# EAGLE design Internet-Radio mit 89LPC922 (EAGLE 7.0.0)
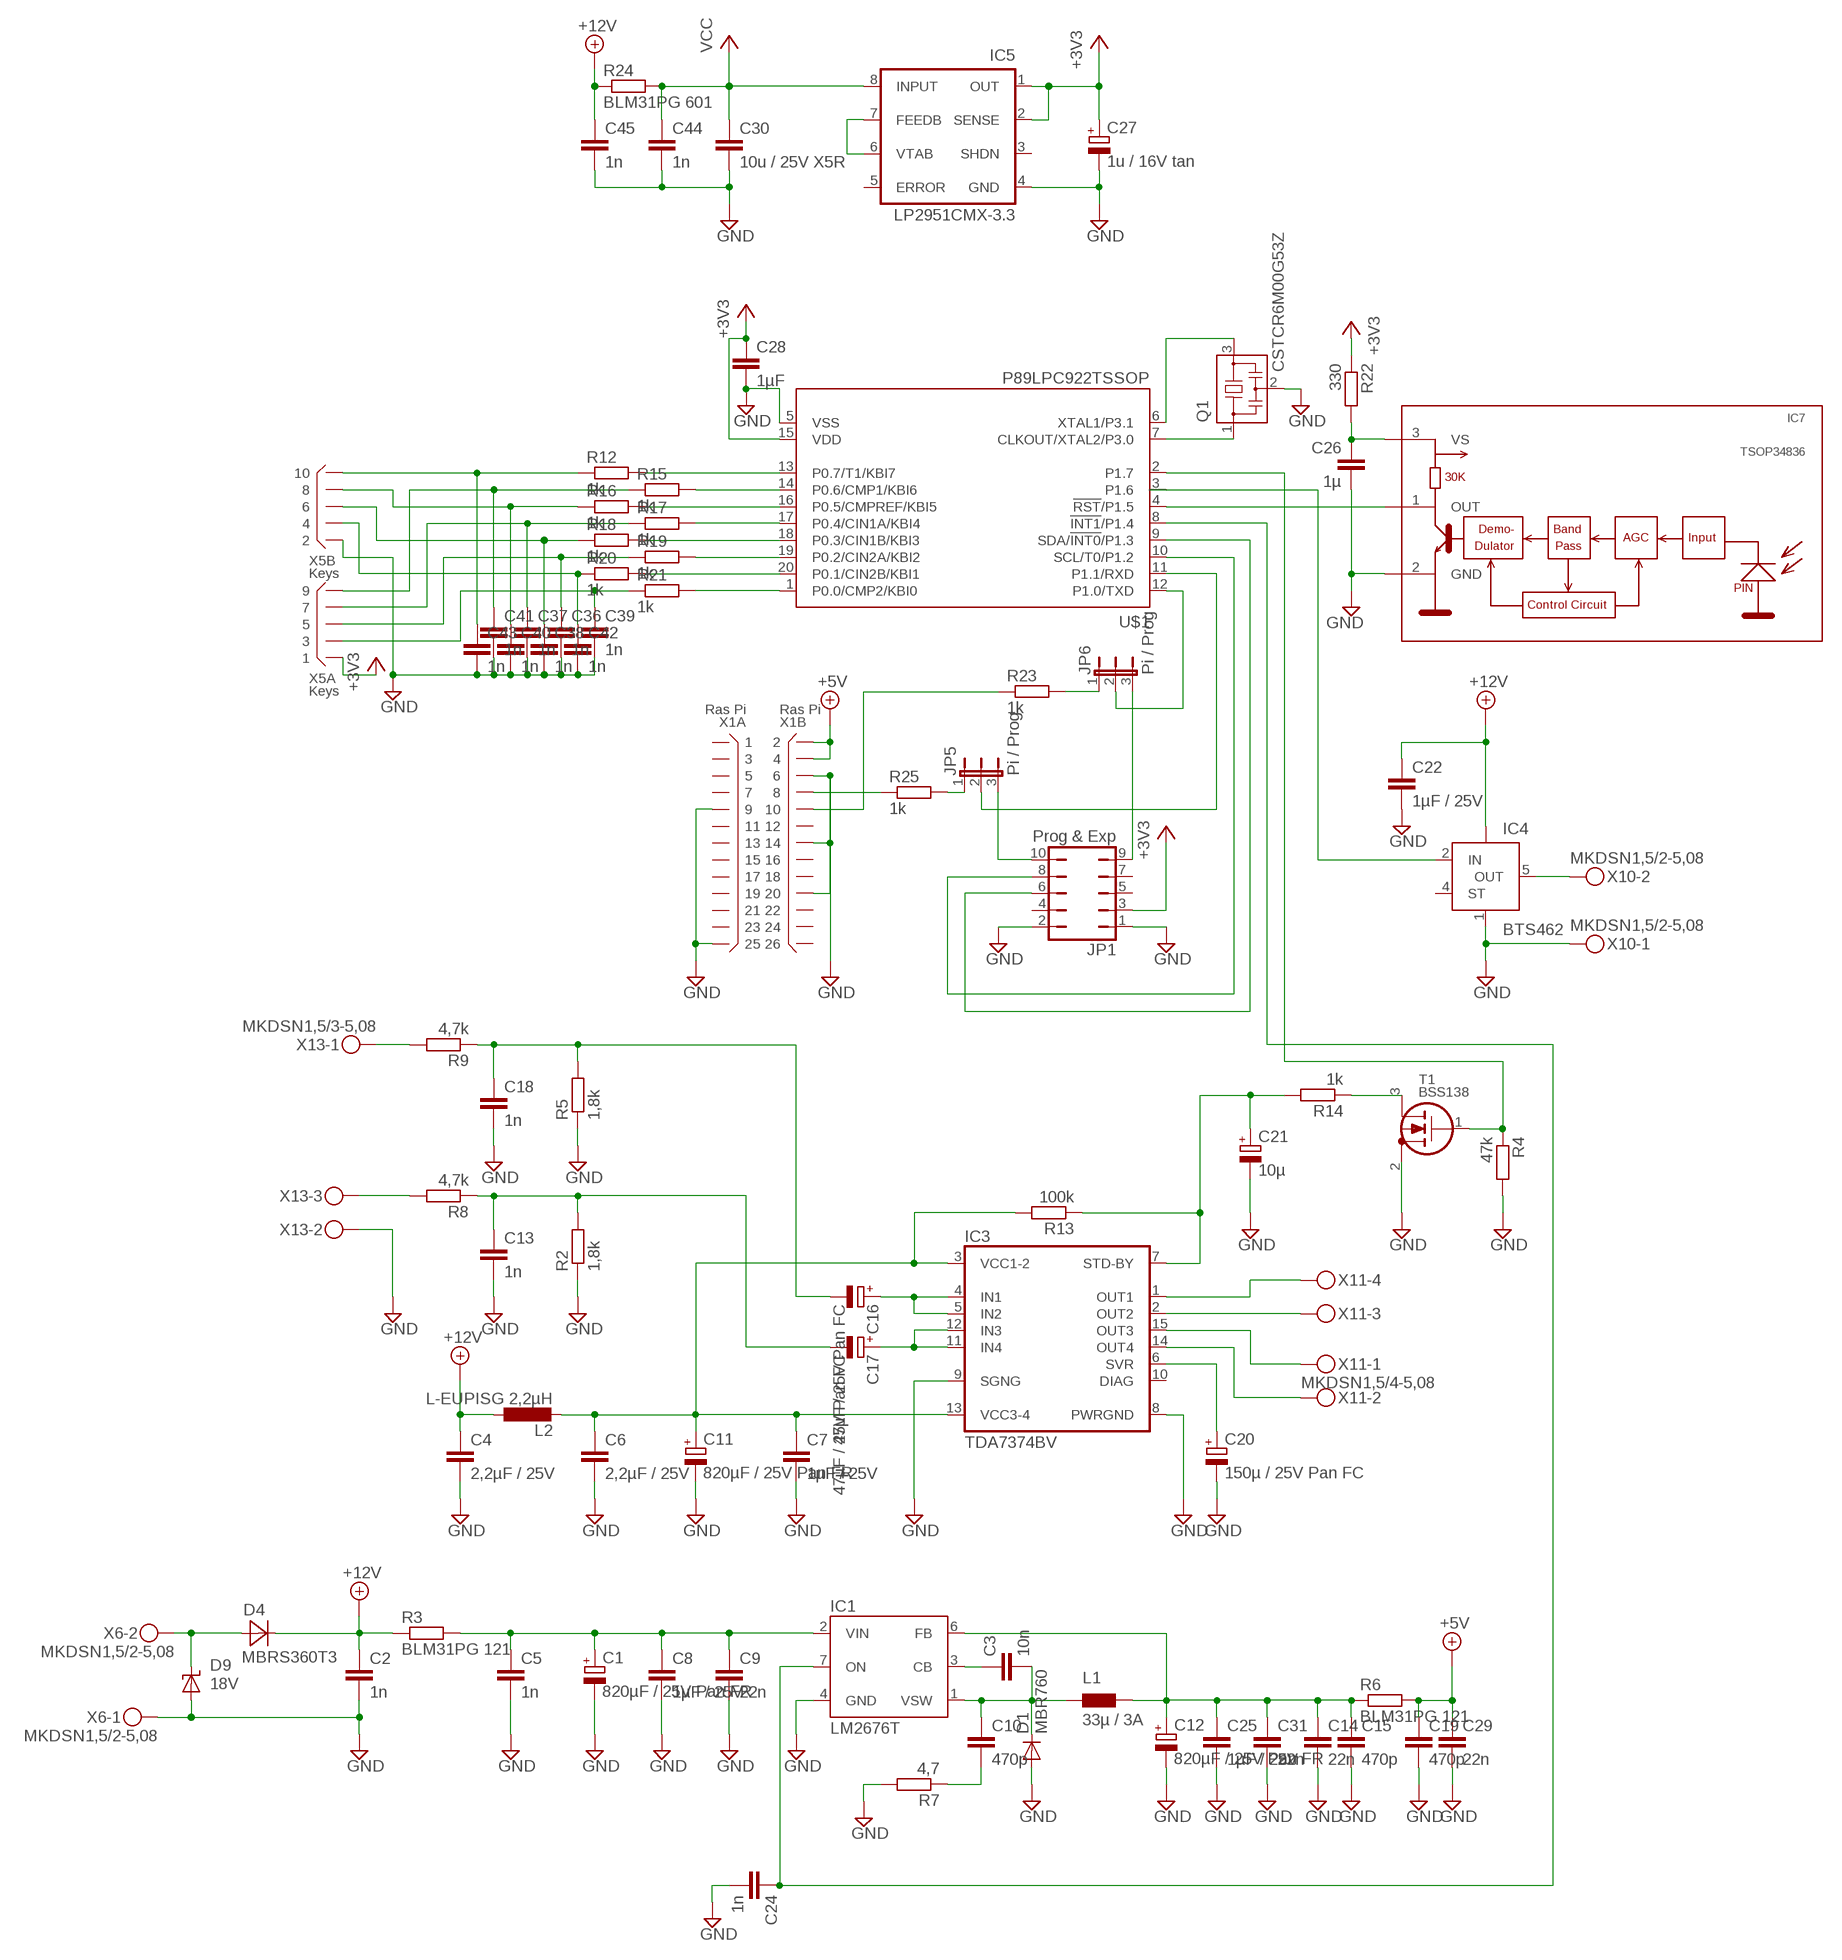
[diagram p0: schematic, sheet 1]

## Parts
C1  820µF / 25V Pan FR  CPOL-EUTT5D10  [TT5D10]
C2  1n  C-EUC0805  [C0805]
C3  10n  C-EUC0805  [C0805]
C4  2,2µF / 25V  C-EUC0805  [C0805]
C5  1n  C-EUC0805  [C0805]
C6  2,2µF / 25V  C-EUC0805  [C0805]
C7  1µF / 25V  C-EUC0805  [C0805]
C8  1µF / 25V  C-EUC0805  [C0805]
C9  22n  C-EUC0805  [C0805]
C10  470p  C-EUC0805  [C0805]
C11  820µF / 25V Pan FR  CPOL-EUTT5D10  [TT5D10]
C12  820µF / 25V Pan FR  CPOL-EUTT5D10  [TT5D10]
C13  1n  C-EUC0805  [C0805]
C14  22n  C-EUC0805  [C0805]
C15  470p  C-EUC0805  [C0805]
C16  47µF / 25V Pan FC  CPOL-EUE2.5-5  [E2,5-5]
C17  47µF / 25V Pan FC  CPOL-EUE2.5-5  [E2,5-5]
C18  1n  C-EUC0805  [C0805]
C19  470p  C-EUC0805  [C0805]
C20  150µ / 25V Pan FC  CPOL-EUE3.5-8  [E3,5-8]
C21  10µ  CPOL-EUE2.5-5  [E2,5-5]
C22  1µF / 25V  C-EUC0805  [C0805]
C24  1n  C-EUC0805  [C0805]
C25  1µF / 25V  C-EUC0805  [C0805]
C26  1µ  C-EUC0805  [C0805]
C27  1u / 16V tan  CPOL-EUCT3216  [CT3216]
C28  1µF  C-EUC0805  [C0805]
C29  22n  C-EUC0805  [C0805]
C30  10u / 25V X5R  C-EUC1206  [C1206]
C31  22n  C-EUC0805  [C0805]
C36  1n  C-EUC0603  [C0603]
C37  1n  C-EUC0603  [C0603]
C38  1n  C-EUC0603  [C0603]
C39  1n  C-EUC0603  [C0603]
C40  1n  C-EUC0603  [C0603]
C41  1n  C-EUC0603  [C0603]
C42  1n  C-EUC0603  [C0603]
C43  1n  C-EUC0603  [C0603]
C44  1n  C-EUC0805  [C0805]
C45  1n  C-EUC0805  [C0805]
D1  MBR760  DIODE-TO220V  [TO220ACS]
D4  MBRS360T3  [SMC]
D9  18V  SUPPRESSOR-SMBJ  [SMBJ]
IC1  LM2676T  [TO220-7]
IC3  TDA7374BV  [MULTIWATT-15V]
IC4  BTS462  BTS428L2  [TO252-5-11]
IC5  LP2951CMX-3.3  [SO-08]
IC7  TSOP34836  [TSOP348]
JP1  Prog & Exp  JP5Q  [JP5Q]
JP5  Pi / Prog  JP2E  [JP2]
JP6  Pi / Prog  JP2E  [JP2]
L1  33µ / 3A  PIS4728  [PIS4728]
L2  L-EUPISG 2,2µH  L-EUPISG  [PISG]
Q1  CSTCR6M00G53Z  [CSTCR6M]
R2  1,8k  R-EU_R1206  [R1206]
R3  BLM31PG 121  R-EU_R1206  [R1206]
R4  47k  R-EU_R1206  [R1206]
R5  1,8k  R-EU_R1206  [R1206]
R6  BLM31PG 121  R-EU_R1206  [R1206]
R7  4,7  R-EU_R1206  [R1206]
R8  4,7k  R-EU_R1206  [R1206]
R9  4,7k  R-EU_R1206  [R1206]
R12  1k  R-EU_R1206  [R1206]
R13  100k  R-EU_R1206  [R1206]
R14  1k  R-EU_R1206  [R1206]
R15  1k  R-EU_R1206  [R1206]
R16  1k  R-EU_R1206  [R1206]
R17  1k  R-EU_R1206  [R1206]
R18  1k  R-EU_R1206  [R1206]
R19  1k  R-EU_R1206  [R1206]
R20  1k  R-EU_R1206  [R1206]
R21  1k  R-EU_R1206  [R1206]
R22  330  R-EU_R1206  [R1206]
R23  1k  R-EU_R1206  [R1206]
R24  BLM31PG 601  R-EU_R1206  [R1206]
R25  1k  R-EU_R1206  [R1206]
T1  BSS138  [SOT23]
U$1  P89LPC922TSSOP  [SOT360]
X1  Ras Pi  X13X2  [X26N-IDC]
X5  Keys  X05X2  [X10N-IDC]
X6  MKDSN1,5/2-5,08  [MKDSN1,5/2-5,08]
X10  MKDSN1,5/2-5,08  [MKDSN1,5/2-5,08]
X11  MKDSN1,5/4-5,08  [MKDSN1,5/4-5,08]
X13  MKDSN1,5/3-5,08  [MKDSN1,5/3-5,08]

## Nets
+3V3: C27.+ C28.1 IC5.1(OUT) IC5.2(SENSE) JP1.3 R22.1 U$1.15(VDD) X5.1
+5V: C19.1 C29.1 R6.2 X1.2 X1.4
+12V: C2.1 C4.1 C22.1 C45.1 D4.C IC4.TAB(VBB) L2.1 R3.1 R24.1
GND: C1.- C2.2 C4.2 C5.2 C6.2 C7.2 C8.2 C9.2 C11.- C12.- C13.2 C14.2 C15.2 C18.2 C19.2 C20.- C21.- C22.2 C24.2 C25.2 C26.2 C27.- C28.2 C29.2 C30.2 C31.2 C36.2 C37.2 C38.2 C39.2 C40.2 C41.2 C42.2 C43.2 C44.2 C45.2 D1.A D9.A IC1.4(GND) IC3.8(PWRGND) IC3.9(SGNG) IC4.1(GND) IC5.4(GND) IC7.2(GND) JP1.1 JP1.2 Q1.2 R2.1 R4.2 R5.1 R7.2 T1.2(S) U$1.5(VSS) X1.6 X1.9 X1.14 X1.20 X1.25 X5.2 X6.1 X10.1 X13.2
N$1: C1.+ C5.1 C8.1 C9.1 IC1.2(VIN) R3.2
N$2: C3.2 C10.1 D1.C IC1.1(VSW) L1.P$1
N$3: IC3.1(OUT1) X11.4
N$4: C3.1 IC1.3(CB)
N$5: IC3.2(OUT2) X11.3
N$6: IC3.15(OUT3) X11.1
N$7: IC3.14(OUT4) X11.2
N$8: C6.1 C7.1 C11.+ IC3.3(VCC1-2) IC3.13(VCC3-4) L2.2 R13.2
N$9: D4.A D9.C X6.2
N$10: C20.+ IC3.6(SVR)
N$11: JP1.10 JP5.3
N$12: C16.- C18.1 R5.2 R9.1
N$13: R9.2 X13.1
N$14: C13.1 C17.- R2.2 R8.1
N$15: C10.2 R7.1
N$16: R8.2 X13.3
N$17: C12.+ C14.1 C15.1 C25.1 C31.1 IC1.6(FB) L1.P$2 R6.1
N$18: C21.+ IC3.7(STD-BY) R13.1 R14.2
N$19: Q1.3 U$1.6(XTAL1/P3.1)
N$20: IC4.5(OUT) X10.2
N$21: Q1.1 U$1.7(CLKOUT/XTAL2/P3.0)
N$22: R21.2 U$1.1(P0.0/CMP2/KBI0)
N$23: R14.1 T1.3(D)
N$24: C16.+ IC3.4(IN1) IC3.5(IN2)
N$25: R4.1 T1.1(G) U$1.2(P1.7)
N$26: C17.+ IC3.11(IN4) IC3.12(IN3)
N$27: R19.2 U$1.19(P0.2/CIN2A/KBI2)
N$28: C24.1 IC1.7(ON) U$1.8(!INT1!/P1.4)
N$29: JP5.2 U$1.11(P1.1/RXD)
N$30: R17.2 U$1.17(P0.4/CIN1A/KBI4)
N$31: R15.2 U$1.14(P0.6/CMP1/KBI6)
N$32: R12.2 U$1.13(P0.7/T1/KBI7)
N$33: IC7.1(OUT) U$1.4(!RST!/P1.5)
N$34: R16.2 U$1.16(P0.5/CMPREF/KBI5)
N$35: R18.2 U$1.18(P0.3/CIN1B/KBI3)
N$36: R20.2 U$1.20(P0.1/CIN2B/KBI1)
N$37: JP6.2 U$1.12(P1.0/TXD)
N$38: JP1.8 U$1.10(SCL/T0/P1.2)
N$39: JP1.6 U$1.9(SDA/!INT0!/P1.3)
N$40: C26.1 IC7.3(VS) R22.2
N$41: IC5.6(VTAB) IC5.7(FEEDB)
N$42: C38.1 R18.1 X5.6
N$43: C36.1 R19.1 X5.5
N$44: C42.1 R20.1 X5.4
N$45: C39.1 R21.1 X5.3
N$46: C43.1 R12.1 X5.10
N$47: C41.1 R15.1 X5.9
N$48: C40.1 R16.1 X5.8
N$49: C37.1 R17.1 X5.7
N$51: JP5.1 R25.2
N$53: JP6.1 R23.2
N$54: R23.1 X1.10
N$55: R25.1 X1.8
N$58: IC4.2(IN) U$1.3(P1.6)
P1.0: JP1.9 JP6.3
VCC: C30.1 C44.1 IC5.8(INPUT) R24.2
Unconnected: IC3.10(DIAG) IC4.4(ST) IC5.3(SHDN) IC5.5(ERROR) JP1.4 JP1.5 JP1.7 X1.1 X1.3 X1.5 X1.7 X1.11 X1.12 X1.13 X1.15 X1.16 X1.17 X1.18 X1.19 X1.21 X1.22 X1.23 X1.24 X1.26

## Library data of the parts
C1 C11 C12 C16 C17 C20 C21 C27 = rcl:CPOL-EU: POLARIZED CAPACITOR, European symbol
C2-C10 C13-C15 C18 C19 C22 C24-C26 C28-C31 C36-C45 = rcl:C-EU: CAPACITOR, European symbol
D1 = diode:DIODE-: DIODE
D4 = diode:MBRS360T3: Surface Mount Schottky Power Rectifier
D9 = diode:SUPPRESSOR-: Suppressor diode
IC1 = v-reg-3:LM2676: National Semiconductor 3.0A "Simple Switcher"(c) 260kHz, Vout 1.2-37V, Vin 40V, 150mOhm DMOS switch, 50µA standby current
IC3 = st-tda737X:TDA7374B
IC4 = infineon:BTS428L2: Smart High-Side Power Switch One Channel: 60mOhm Status Feedback Source: Source: www.infineon.com .. BTS428L2_20030912.pdf; OC_FARNELL: unknown; OC_NEWARK: unknown
IC5 = v-reg:LP2951?*: Series of Adjustable Micropower Voltage Regulators Source: http://cache.national.com/ds/LP/LP2950.pdf
IC7 = vishay-1:TSOP348*: IR Receiver Modules for Remote Control Systems http://www.vishay.com/ir-receiver-modules/
JP1 = jumper:JP5Q: JUMPER
JP5 JP6 = jumper:JP2E: JUMPER
L1 = inductor-fastron:PIS4728: Fastron SMD Power Inductors
L2 = Inductor-Fastron (2):L-EU
Q1 = murata-filter:CSTCR: Resonator Source: murata.co.jp; MPN: CSTCR6M00G53-R0; OC_FARNELL: 1170434; OC_NEWARK: 25M8759
R2 R4 R5 R7-R9 R13 R14 R22 R23 R25 = rcl:R-EU_: RESISTOR, European symbol
R3 R6 R12 R15-R21 R24 = resistor:R-EU_: RESISTOR, European symbol
T1 = transistors:BSS138: BSS138: N-channel enhancement MOSFET (ON Semiconductor) 50V Uds, 200mA Id, 225mW Ptot, 3.5&Omega; Rdson
U$1 = 89LPC922:P89LPC922
X1 = connectors:X13X2: Connector 2x13 pins
X5 = connectors:X05X2: Connector 2x5 pins
X6 X10 = con-phoenix-508:MKDSN1,5/2-5,08: MKDSN 1,5/ 2-5,08 Printklemme; MPN: MKDSN 1,5/2-5.08; OC_FARNELL: 1792903; OC_NEWARK: 30M2397
X11 = con-phoenix-508:MKDSN1,5/4-5,08: MKDSN 1,5/ 4-5,08 Printklemme Nennstrom: 13,5 A Nennspannung: 250 V Rastermaß: 5,08 mm Polzahl: 4 Anschlussart: Schraubanschluss Montage: Löten Anschlussrichtung Leiter/Platine: 0 ° Artikelnummer: 1729144 Source: http://eshop.phoenixcontact.com .. 1729144.pdf
X13 = con-phoenix-508:MKDSN1,5/3-5,08: MKDSN 1,5/ 3-5,08 Printklemme Nennstrom: 13,5 A Nennspannung: 250 V Rastermaß: 5,08 mm Polzahl: 3 Anschlussart: Schraubanschluss Montage: Löten Anschlussrichtung Leiter/Platine: 0 ° Artikelnummer: 1729131 Source: http://eshop.phoenixcontact.com .. 1729131.pdf; MPN: SMKDSN1,5/3-5,08; OC_FARNELL: 1792904; OC_NEWARK: 70R0299

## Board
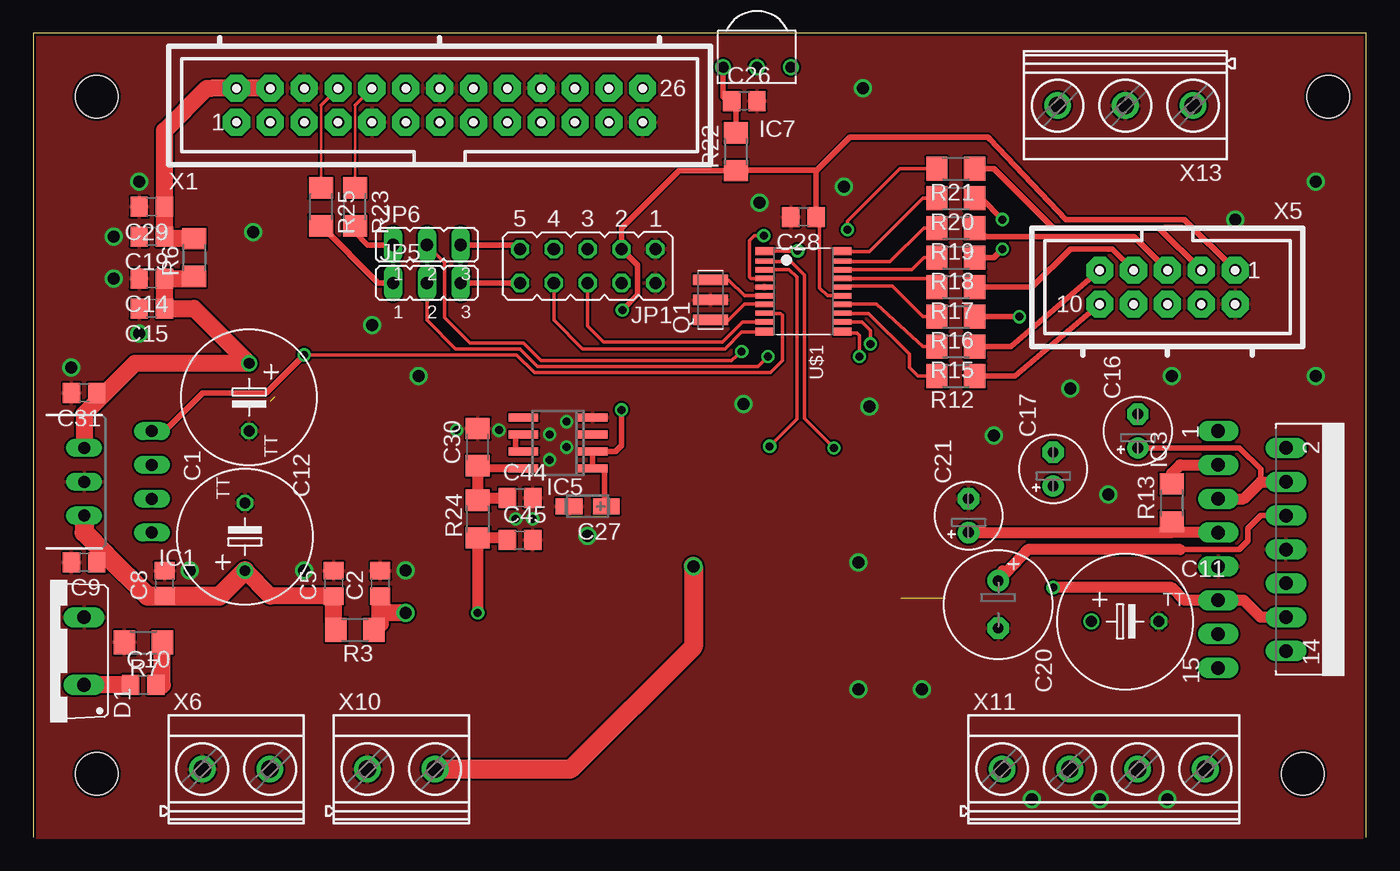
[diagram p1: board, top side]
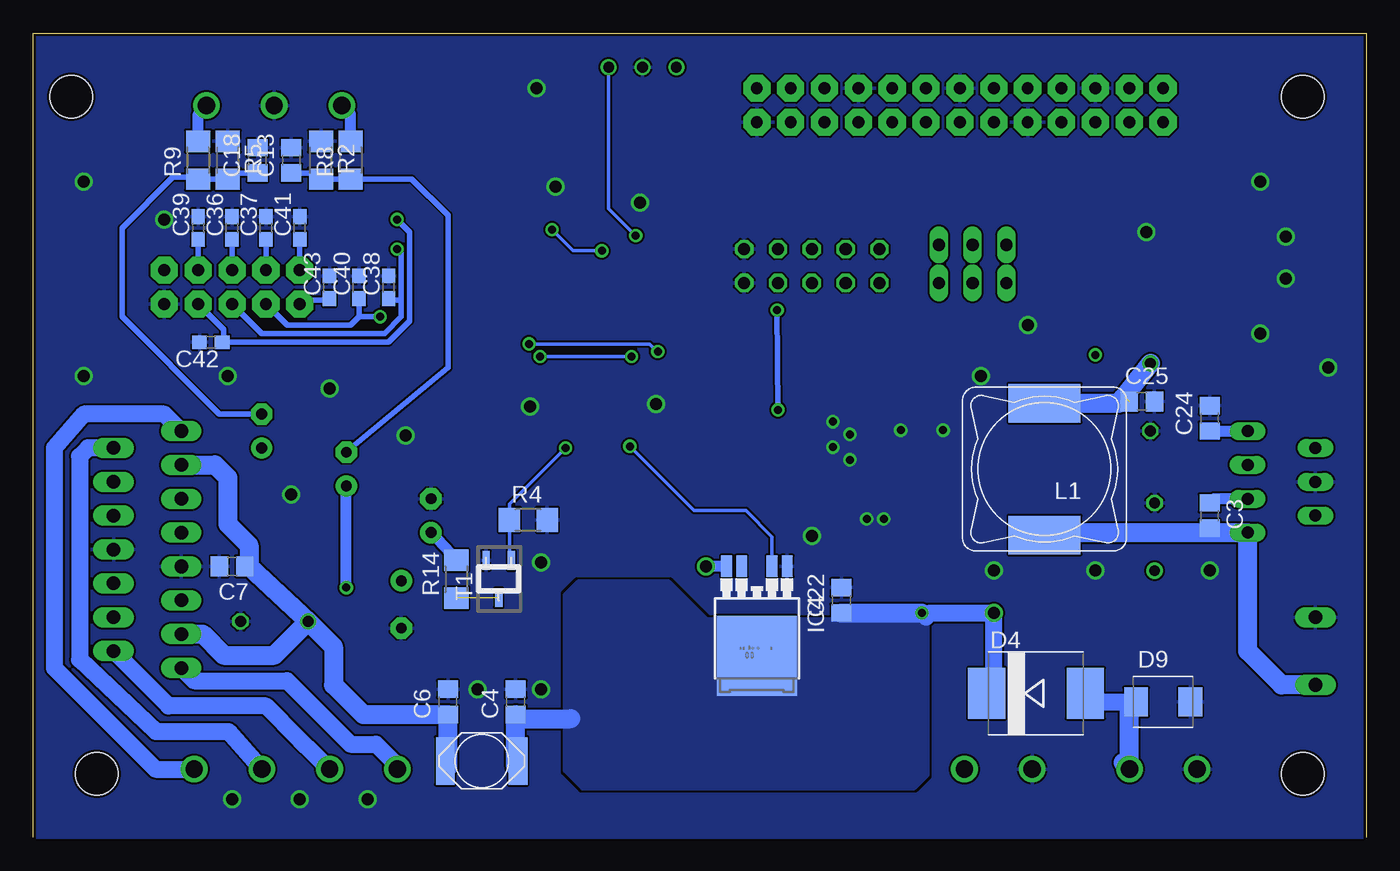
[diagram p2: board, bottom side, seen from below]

Size 100 x 60.33 mm. Coordinates in mm from the lower left corner, seen from the top.
Outline: 100,0 100,60.33 0,60.33 0,0
Copper layers (1*16): Top 0.035mm / dielectric 1.5mm / Bottom 0.035mm
Design rules "platinensammler_02": minimum track width 0.15mm, minimum drill 0.3mm, track to track 0.15mm, track to pad 0.15mm, pad to pad 0.15mm, via to via 0.15mm, smd to smd 0mil, copper to edge 0.2mm, drill to drill 0.2mm, minimum pad ring 0.2mm, minimum via ring 0.2mm, stop-mask expansion 4mil, vias tented up to drill 0.8mm, thermal gap 0.15mm
Holes 3.2 mm at 4.76,4.76 4.76,55.56 97.16,55.56 95.25,4.76

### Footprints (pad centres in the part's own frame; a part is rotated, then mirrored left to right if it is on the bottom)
TT5D10 = drill 0.813: + -2.54,0 | drill 0.813 octagon: - 2.54,0
C0805 = smd 1.3 x 1.5: 1 -0.95,0; 2 0.95,0
E2,5-5 = drill 0.813 pad 1.6: + -1.27,0 | drill 0.813 pad 1.6 octagon: - 1.27,0
E3,5-8 = drill 0.813 pad 1.6: + -1.778,0 | drill 0.813 pad 1.6 octagon: - 1.778,0
CT3216 = smd 2 x 1.2: + -1.4,0; - 1.4,0
C1206 = smd 1.6 x 1.8: 1 -1.4,0; 2 1.4,0
C0603 = smd 1.1 x 1: 1 -0.85,0; 2 0.85,0
TO220ACS = drill 1.016 long: A 2.54,-2.54; C -2.54,-2.54
SMC = smd 2.8 x 3.8: A 3.7,0; C -3.7,0
SMBJ = smd 1.78 x 2.16: A 2.04,0; C -2.03,0
TO220-7 = drill 0.9 long: 1 -3.81,-5.08; 2 -2.54,0; 3 -1.27,-5.08; 4 0,0; 5 1.27,-5.08; 6 2.54,0; 7 3.81,-5.08
MULTIWATT-15V = drill 1.016 long: 1 -8.89,-7.62; 2 -7.62,-2.54; 3 -6.35,-7.62; 4 -5.08,-2.54; 5 -3.81,-7.62; 6 -2.54,-2.54; 7 -1.27,-7.62; 8 0,-2.54; 9 1.27,-7.62; 10 2.54,-2.54; 11 3.81,-7.62; 12 5.08,-2.54; 13 6.35,-7.62; 14 7.62,-2.54; 15 8.89,-7.62
TO252-5-11 = smd 0.8 x 1.6: 1 -2.28,-5.41; 2 -1.14,-5.41; 4 1.14,-5.41; 5 2.28,-5.41 | smd 6 x 6: TAB 0,1.3
SO-08 = smd 0.6 x 2.2: 1 -1.905,-2.6; 2 -0.635,-2.6; 3 0.635,-2.6; 4 1.905,-2.6; 5 1.905,2.6; 6 0.635,2.6; 7 -0.635,2.6; 8 -1.905,2.6
TSOP348 = drill 0.8: 1 -2.54,0; 2 0,0; 3 2.54,0
JP5Q = drill 0.914 octagon: 1 -5.08,-1.27; 2 -5.08,1.27; 3 -2.54,-1.27; 4 -2.54,1.27; 5 0,-1.27; 6 0,1.27; 7 2.54,-1.27; 8 2.54,1.27; 9 5.08,-1.27; 10 5.08,1.27
JP2 = drill 0.914 long: 1 -2.54,0; 2 0,0; 3 2.54,0
PIS4728 = smd 5.4 x 2.9: P$1 0,4.95; P$2 0,-4.95
PISG = smd 1.4 x 3.56: 1 -2.73,0; 2 2.73,0
CSTCR6M = smd 0.8 x 2.6: 1 -1.5,0; 2 0,0; 3 1.5,0
R1206 = smd 1.6 x 1.803: 1 -1.422,0; 2 1.422,0
SOT23 = smd 0.55 x 1.4: 1 0.95,1.4; 2 -0.95,1.4; 3 0,-1.4
SOT360 = smd 0.6 x 1.35: 1 -3.025,-2.925; 10 3.025,-2.925; 11 3.025,2.925; 20 -3.025,2.925 | smd 0.4 x 1.35: 2 -2.275,-2.925; 3 -1.625,-2.925; 4 -0.975,-2.925; 5 -0.325,-2.925; 6 0.325,-2.925; 7 0.975,-2.925; 8 1.625,-2.925; 9 2.275,-2.925; 12 2.275,2.925; 13 1.625,2.925; 14 0.975,2.925; 15 0.325,2.925; 16 -0.325,2.925; 17 -0.975,2.925; 18 -1.625,2.925; 19 -2.275,2.925
X26N-IDC = drill 0.889 pad 2.032 octagon: 1 -15.24,-1.27; 2 -15.24,1.27; 3 -12.7,-1.27; 4 -12.7,1.27; 5 -10.16,-1.27; 6 -10.16,1.27; 7 -7.62,-1.27; 8 -7.62,1.27; 9 -5.08,-1.27; 10 -5.08,1.27; 11 -2.54,-1.27; 12 -2.54,1.27; 13 0,-1.27; 14 0,1.27; 15 2.54,-1.27; 16 2.54,1.27; 17 5.08,-1.27; 18 5.08,1.27; 19 7.62,-1.27; 20 7.62,1.27; 21 10.16,-1.27; 22 10.16,1.27; 23 12.7,-1.27; 24 12.7,1.27; 25 15.24,-1.27; 26 15.24,1.27
X10N-IDC = drill 0.889 pad 2.032 octagon: 1 -5.08,-1.27; 2 -5.08,1.27; 3 -2.54,-1.27; 4 -2.54,1.27; 5 0,-1.27; 6 0,1.27; 7 2.54,-1.27; 8 2.54,1.27; 9 5.08,-1.27; 10 5.08,1.27
MKDSN1,5/2-5,08 = drill 1.3 pad 2: 1 -2.561,0.025; 2 2.519,0.025
MKDSN1,5/4-5,08 = drill 1.3 pad 2: 1 -7.641,0.025; 2 -2.561,0.025; 3 2.519,0.025; 4 7.599,0.025
MKDSN1,5/3-5,08 = drill 1.3 pad 2: 1 -7.641,0.025; 2 -2.561,0.025; 3 2.519,0.025

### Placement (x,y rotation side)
C1  15.88,22.54 90 top
C2  26.04,19.05 90 top
C3  11.75,24.13 270 bottom
C4  63.82,10.16 90 bottom
C5  22.54,19.05 90 top
C6  68.9,10.16 90 bottom
C7  85.09,20.32 180 bottom
C8  9.84,19.05 90 top
C9  3.81,20.64 180 top
C10  8.26,11.43 0 top
C11  81.92,16.19 0 top
C12  16.19,33.02 270 top
C13  80.64,50.8 90 bottom
C14  8.89,41.91 180 top
C15  8.89,39.69 180 top
C16  82.87,30.48 90 top
C17  76.52,27.62 90 top
C18  83.19,50.8 90 bottom
C19  8.89,45.09 180 top
C20  72.39,17.46 270 top
C21  70.17,24.13 90 top
C22  39.37,17.78 90 bottom
C24  11.75,31.43 90 bottom
C25  16.83,32.7 0 bottom
C26  53.34,55.24 0 top
C27  41.59,24.83 180 top
C28  57.78,46.55 180 top
C29  8.89,47.31 180 top
C30  33.34,29.27 90 top
C31  3.81,33.34 180 top
C36  85.09,45.72 90 bottom
C37  82.55,45.72 90 bottom
C38  73.34,41.27 90 bottom
C39  87.63,45.72 90 bottom
C40  75.56,41.27 90 bottom
C41  80.01,45.72 90 bottom
C42  86.68,37.15 180 bottom
C43  77.79,41.27 90 bottom
C44  36.51,25.46 0 top
C45  36.51,22.29 0 top
D1  1.27,13.97 90 top
D4  24.77,10.79 0 bottom
D9  15.24,10.16 0 bottom
IC1  3.81,26.67 90 top
IC3  96.52,21.59 270 top
IC4  45.72,14.92 180 bottom
IC5  39.37,29.59 90 top
IC7  54.29,57.78 180 top
JP1  41.59,42.86 180 top
JP5  29.53,41.59 0 top
JP6  29.53,44.45 0 top
L1  24.13,27.62 180 bottom
L2  66.36,5.71 180 bottom
Q1  50.8,40.32 90 top
R2  78.42,50.8 270 bottom
R3  24.13,15.56 180 top
R4  62.87,23.81 0 bottom
R5  85.41,50.8 270 bottom
R6  12.06,43.5 90 top
R7  8.26,14.61 180 top
R8  76.2,50.8 90 bottom
R9  87.63,50.8 90 bottom
R12  69.22,34.61 180 top
R13  85.41,25.08 90 top
R14  68.26,19.37 90 bottom
R15  69.22,36.83 180 top
R16  69.22,39.05 180 top
R17  69.22,41.27 180 top
R18  69.22,43.5 180 top
R19  69.22,45.72 180 top
R20  69.22,47.94 180 top
R21  69.22,50.16 180 top
R22  52.7,51.44 90 top
R23  24.13,47.31 270 top
R24  33.34,23.88 90 top
R25  21.59,47.31 270 top
T1  65.09,19.37 0 bottom
U$1  57.78,40.96 270 top
X1  30.48,54.93 0 top
X5  85.09,41.27 180 top
X6  15.24,5.08 0 top
X10  27.62,5.08 0 top
X11  80.33,5.08 0 top
X13  79.38,54.93 180 top

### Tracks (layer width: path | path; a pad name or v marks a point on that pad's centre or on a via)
+3V3  (via drill 0.6)
  Top 0.254: U$1.15 59.56,40.64 58.99,41.21 58.99,46.16 58.99,46.29 C28.1
  Top 0.406: 43.18,24.83 C27.+ 42.86,25.46 42.86,27.69 IC5.1 IC5.2 43.69,28.96 44.13,29.4 v44.13,32.07 | X5.1 86.36,46.35 77.47,46.35 71.75,52.39 71.63,52.51 61.28,52.51 58.8,50.04 58.74,50.04 | 58.74,50.04 52.73,50.04 R22.1 48.42,50.01 44.13,45.72 JP1.3 45.34,42.93 45.34,40.7 v44.2,39.56 | 58.74,50.04 58.73,50.03 C28.1
  Bottom 0.406: v44.13,32.07 v44.2,39.56
+5V
  Top 1.27: X1.4 X1.2 13.34,56.2 13.02,56.2 9.84,53.02 C29.1 C19.1 10.01,44.92 R6.2
+12V  (via drill 0.6, 0.9)
  Top 0.813: v33.34,16.83 R24.1 35.4,22.45 C45.1
  Top 1.27: R3.1 26.04,16.04 26.04,16.83 | 26.04,16.83 C2.1 | v27.94,16.83 26.04,16.83
  Bottom 0.813: v33.34,16.83 33.02,16.51 | L2.1 63.82,5.27 | C4.1 63.5,8.89
  Bottom 1.27: 33.02,16.51 32.7,16.83 v27.94,16.83 27.94,11.32 D4.C
  Bottom 1.422: C22.1 v33.34,16.83 | 63.82,5.27 C4.1 | 63.5,8.89 59.69,8.89
  pour Bottom (no thermals): 38.42,16.83 39.05,16.19 49.53,16.19 52.39,19.05 59.05,19.05 60.01,18.1 60.01,5.08 58.74,3.81 33.97,3.81 33.02,4.76 33.02,16.83
GND  (via drill 0.6, 0.9)
  other vias: 61.91,11.11 66.67,11.11 20.32,20 27.94,20 80.01,2.86 85.09,2.86 74.93,2.86 53.28,32.51 96.2,34.61 96.2,49.21 61.91,20.64 77.79,33.66 16.51,45.4 40.01,31.18 38.73,30.23 38.73,28.32 40.01,29.27 36.2,23.88 37.47,23.88 28.89,34.61 72.07,30.16 41.59,22.61 31.75,30.54 25.4,38.42 34.92,30.54 85.41,34.61 90.17,46.35 80.64,25.72 7.94,37.78 6.03,41.91 6.03,45.09 7.94,49.21 2.86,35.24 11.75,20 62.74,32.32 62.23,56.2 60.83,48.83 54.48,47.62
  pour Bottom (rank 2): 0,0 100.33,0 100.01,60.33 0,60.33
  pour Top: 0,60.33 100.01,60.33 100.33,0 0,0
N$1
  Top 1.27: R3.2 22.54,16.03 C5.1 17.78,18.1 C1.+ | C9.1 5.4,21.27
  Top 1.422: IC1.2 3.81,22.86 5.4,21.27 8.57,18.1 C8.1 11.43,18.1 13.97,18.1 C1.+
N$2
  Top 1.27: C10.1 D1.C
  Bottom 0.813: C3.2 11.43,22.86 IC1.1
  Bottom 1.422: D1.C 6.35,11.43 8.89,13.97 IC1.1 24,22.86 L1.P$1
N$3
  Bottom 1.27: IC3.1 90.17,31.75 96.2,31.75 98.42,29.21 98.42,12.7 90.83,5.11 X11.4
N$4
  Bottom 0.406: 11.43,25.4
  Bottom 0.813: IC1.3 11.43,25.4 | C3.1 11.43,25.4
N$5
  Bottom 1.27: X11.3 85.36,7.94 90.81,7.94 96.52,13.34 96.52,28.57 95.89,29.21 IC3.2
N$6
  Bottom 1.27: IC3.15 87.95,11.75 80.96,11.75 76.2,6.99 74.3,6.99 72.71,5.4 72.71,5.08 | X11.1 72.71,5.08 | 72.71,5.08
N$7
  Bottom 1.27: X11.2 77.79,5.13 80.01,7.3 82.55,9.84 89.85,9.84 IC3.14
N$8
  Top 0.813: R13.2 85.41,27.3 86.04,27.94 IC3.3
  Bottom 0.813: L2.2 68.9,5.27 | C7.1 83.82,20.32
  Bottom 1.422: 68.9,5.27 C6.1 75.25,9.21 77.47,11.43 77.47,14.29 C11.+ | IC3.3 86.36,27.94 85.41,26.99 85.41,23.5 83.82,21.91 83.82,20.32 C11.+ | IC3.13 87.31,15.24 85.72,13.65 81.92,13.65 C11.+
N$9
  Bottom 1.27: D4.A 20.43,10.16 D9.C
  Bottom 1.422: X6.2 17.78,5.13 | 17.78,5.13 17.78,9.84 17.46,10.16 D9.C 17.14,10.16 | 17.78,5.13 18.24,5.59
N$10
  Top 0.406: IC3.6 92.08,24.13 91.12,23.18 91.12,22.23 90.49,21.59 86.04,21.59
  Top 0.813: 86.04,21.59 74.61,21.59 C20.+ 72.71,20
N$11
  Top 0.406: JP1.10 JP5.3
N$12
  Bottom 0.406: C18.1 84.94,49.85 R5.2 R9.1 87.78,49.53 89.53,49.53 93.34,45.72 93.34,39.05 86.04,31.75 C16.-
N$13
  Bottom 0.813: R9.2 87.63,54.29 X13.1
N$14
  Bottom 0.406: C13.1 78.89,49.85 R2.2 R8.1 71.6,49.38 68.9,46.67 68.9,35.24 C17.-
N$15
  Top 1.27: C10.2 9.68,11.43 R7.1
N$16
  Bottom 0.813: R8.2 76.2,54.29 76.81,54.9 X13.3
N$17  (1 unrouted)
  Top 1.27: 4.76,32.7 7.62,35.56 C12.+ 12.06,39.69 C15.1 C14.1 11.9,41.91 R6.1 | IC1.6 3.81,31.75 4.76,32.7 | C31.1 4.76,32.7
  Bottom 0.813: 18.1,33.02 18.19,33.02
  Bottom 1.422: L1.P$2 18.55,32.57 18.19,33.02 C12.+
N$18
  Top 0.813: C21.+ 85.41,22.86 | 85.41,22.86 R13.1 | IC3.7 85.41,22.86
  Bottom 0.813: C21.+ R14.2
N$19
  Top 0.254: U$1.6 53.34,40.64 52.16,41.82 Q1.3
N$20  (via drill 0.9)
  Top 1.422: v49.53,20.32 49.53,14.29 40.3,5.1 X10.2
  Bottom 0.813: IC4.5 48.3,20.32 v49.53,20.32
N$21
  Top 0.254: U$1.7 54.84,40.01 53.34,40.01 52.16,38.82 Q1.1
N$22  (via drill 0.6)
  Top 0.254: R21.2 65.02,50.16 61.09,46.23 v61.09,45.59 | v57.34,44.01 57.19,43.98 U$1.1
  Bottom 0.254: v61.09,45.59 59.5,44.01 v57.34,44.01
N$23  (1 unrouted)
N$24
  Top 0.406: C16.+ 90.49,29.21 92.08,27.62 92.08,26.67
  Top 0.813: IC3.5 90.81,25.4 92.08,26.67 IC3.4
N$25  (via drill 0.6)
  Top 0.254: U$1.2 54.91,43.18 56.83,43.18 57.85,42.16 57.85,31.43 v60.07,29.21
  Bottom 0.254: T1.1 64.29,20.92 R4.1 64.29,24.99 v60.07,29.21
N$26  (via drill 0.6)
  Top 0.813: IC3.12 92.08,16.51 90.81,17.78 IC3.11 86.36,17.78 85.41,18.73 v76.52,18.73
  Bottom 0.813: v76.52,18.73 C17.+
N$27
  Top 0.254: U$1.19 60.76,43.18 64.26,43.18 66.8,45.72 R19.2
  Top 0.406: 67.47,45.4 R19.2
N$28  (via drill 0.6)
  Top 0.254: U$1.8 54.89,39.31 56.07,39.31 56.2,39.18 56.2,35.75 55.31,34.86 37.59,34.86 36.26,36.2 v20.32,36.2
  Top 0.406: v20.32,36.2 17.46,33.34 12.7,33.34 9.84,30.48 IC1.7
  Bottom 0.813: C24.1 11.43,30.48 IC1.7
N$29  (via drill 0.6)
  Top 0.254: JP5.2 29.53,38.8 31.69,36.64 36.51,36.64 37.85,35.31 54.36,35.31 v55.12,36.07 | U$1.11 60.8,37.85 61.78,37.85 61.98,37.66 v61.98,36.07
  Bottom 0.254: v61.98,36.07 v55.12,36.07
N$30
  Top 0.254: U$1.17 60.73,41.91 67.18,41.91 67.82,41.27 R17.2
N$31
  Top 0.254: U$1.14 60.73,40.01 63.25,40.01 66.74,36.83 R15.2
N$32
  Top 0.254: U$1.13 60.74,39.31 62.67,39.31 65.72,36.26 65.72,35.24 66.36,34.61 R12.2
N$33  (via drill 0.6)
  Top 0.254: U$1.4 54.84,41.91 53.85,41.91 53.72,42.04 53.72,44.77 54.1,45.15 v54.8,45.15
  Bottom 0.254: v54.8,45.15 56.83,47.18 IC7.1
N$34
  Top 0.254: U$1.16 60.77,41.34 64.45,41.34 66.74,39.05 R16.2
N$35
  Top 0.254: U$1.18 60.74,42.61 65.91,42.61 66.8,43.5 R18.2
N$36
  Top 0.254: U$1.20 60.75,43.94 62.74,43.94 66.74,47.94 R20.2
N$37  (via drill 0.6)
  Top 0.254: JP6.2 30.86,43.12 30.86,38.99 32.77,37.08 36.77,37.08 38.1,35.75 52.39,35.75 v53.15,36.45 | U$1.12 62.17,38.67 62.8,38.04 v62.8,37.02
  Bottom 0.254: v62.8,37.02 53.78,37.02 53.21,36.45 v53.15,36.45
N$38
  Top 0.254: U$1.10 54.84,37.91 53.15,37.91 51.88,36.64 41.21,36.64 39.05,38.8 JP1.8
N$39
  Top 0.254: U$1.9 54.85,38.67 53.21,38.67 51.69,37.15 42.8,37.15 41.59,38.35 JP1.6
N$40
  Top 0.406: R22.2 52.7,54.76 51.75,55.56 | IC7.3 51.75,55.56 | 51.75,55.56 C26.1
N$41
  Top 0.406: IC5.7 36.2,29.02 36.2,30.23 IC5.6
N$42  (via drill 0.6)
  Top 0.406: v72.71,44.13 72.07,43.5 R18.1
  Bottom 0.406: X5.6 82.87,37.78 73.66,37.78 72.39,39.05 72.39,40.32 | 72.39,40.32 72.39,43.81 v72.71,44.13 | C38.1 73.56,40.32 72.39,40.32
N$43
  Top 0.406: X5.5 82.55,45.09 71.44,45.09 70.8,45.72 R19.1
  Bottom 0.406: C36.1 X5.5
N$44  (via drill 0.6)
  Top 0.406: R20.1 71.12,47.94 v72.71,46.35
  Bottom 0.406: v72.71,46.35 71.75,45.4 71.75,38.73 73.34,37.15 85.72,37.15 | X5.4 85.72,38.1 85.72,37.15 | C42.1 85.72,37.15
N$45
  Top 0.406: X5.3 84.45,45.72 76.52,45.72 72.07,50.16 R21.1
  Bottom 0.406: C39.1 X5.3
N$46
  Top 0.406: X5.10 73.66,34.61 R12.1
  Bottom 0.406: X5.10 79.69,40.32 77.79,40.32 C43.1
N$47
  Top 0.406: X5.9 73.34,36.83 R15.1
  Bottom 0.406: X5.9 C41.1
N$48  (via drill 0.6)
  Top 0.406: v73.98,39.05 R16.1
  Bottom 0.406: X5.8 80.96,38.42 76.2,38.42 75.56,39.05 | 75.56,39.05 v73.98,39.05 | C40.1 75.56,39.05
N$49
  Top 0.406: R17.1 74.93,41.27 77.79,44.13 80.96,44.13 X5.7
  Bottom 0.406: C37.1 X5.7
N$51
  Top 0.406: JP5.1 25.88,41.59 R25.2
N$53
  Top 0.406: R23.2 24.13,45.4 25.08,44.45 JP6.1
N$54
  Top 0.203: 24.13,54.93 R23.1
  Top 0.254: X1.10 24.13,54.93
N$55
  Top 0.203: 21.59,54.93 R25.1
  Top 0.254: X1.8 21.59,54.93
N$58  (via drill 0.6)
  Top 0.254: U$1.3 54.96,42.48 55.09,42.61 56.71,42.61 57.28,42.04 57.28,31.37 v55.24,29.34
  Bottom 0.254: v55.24,29.34 50.42,24.51 46.55,24.51 44.58,22.55 IC4.2
P1.0
  Top 0.406: JP6.3 36.2,44.45 JP1.9
VCC
  Top 0.61: IC5.8 33.66,27.69 33.47,27.87 C30.1
  Top 0.813: C30.1 R24.2 33.5,25.46 C44.1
